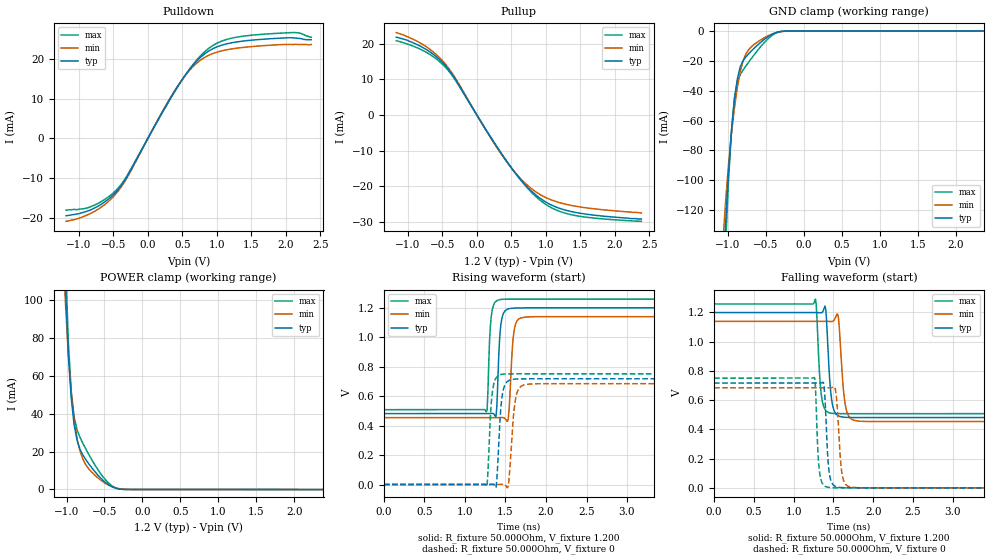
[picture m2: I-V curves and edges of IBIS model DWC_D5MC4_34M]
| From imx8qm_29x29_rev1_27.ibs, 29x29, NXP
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[Model] DWC_D5MC4_34M
Model_type   I/O
Polarity   Non-Inverting
Enable   Active-High
C_comp   1.264pF   1.181pF   1.367pF
C_comp_pullup   284.419fF   263.792fF   311.358fF
C_comp_pulldown 969.046fF   901.845fF   1.049pF
Vinh = 693.000mV
Vinl = 507.000mV
Vmeas = 600.000mV
Vref = 600.000mV
Rref = 50Ohms
Cref = 0pF
[Model Spec]
Vinh   693.000mV   663.000mV   723.000mV
Vinl   507.000mV   477.000mV   537.000mV
Vmeas   600.000mV   570.000mV   630.000mV
Vref   600.000mV   570.000mV   630.000mV
D_overshoot_ampl_h 0.4 NA   NA
D_overshoot_ampl_l 0.4 NA   NA
D_overshoot_area_l 60.000p NA   NA
D_overshoot_area_h 60.000p NA   NA
[Receiver Thresholds]
Vth = 600.000mV
Vth_min = 588.000mV
Vth_max = 612.000mV
Vinh_ac = 68.000mV
Vinh_dc = 68.000mV
Vinl_ac = -68.000mV
Vinl_dc = -68.000mV
Tslew_ac = 5.000ns
Reference_supply Pullup_ref
[Temperature Range]   25.000   125.000   -40.000
[Voltage Range]   1.200V   1.140V   1.260V
[GND Clamp Reference]   0.00V   0.00V   0.00V
[C Comp Corner]
| variable   typ   min   max
C_comp 1.264pF   1.367pF   1.181pF
C_comp_pullup 284.419fF   311.358fF   263.792fF
C_comp_pulldown 969.046fF   1.049pF   901.845fF
[Pulldown Reference]   0.00V   0.00V   0.00V
[POWER Clamp Reference]   1.200V   1.140V   1.260V
[Pullup Reference]   1.200V   1.140V   1.260V
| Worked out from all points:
|   slope of the pulldown table from 0 to 0.18 V, typ, clamps not added: 31.8 ohm
|   slope of the pullup table from 0 to 0.18 V, typ, clamps not added: 31.9 ohm
|   GND clamp passes 1 mA (typ) near -0.36 V on its own axis
|   POWER clamp passes 1 mA (typ) near -0.38 V on its own axis
|   rising waveform, R_fixture 50.000Ohm, V_fixture 1.200: 20-80 % time 37.2ps typ, 43.2ps min, 34.2ps max; typ from 0.481 V to 1.2 V
|   rising waveform, R_fixture 50.000Ohm, V_fixture 0: 20-80 % time 47.7ps typ, 56.6ps min, 43.8ps max; typ from 0 V to 0.717 V
|   falling waveform, R_fixture 50.000Ohm, V_fixture 1.200: 20-80 % time 50.4ps typ, 57.6ps min, 46.1ps max; typ from 1.2 V to 0.481 V
|   falling waveform, R_fixture 50.000Ohm, V_fixture 0: 20-80 % time 41.8ps typ, 50ps min, 36.8ps max; typ from 0.717 V to 0 V
[GND Clamp]
-1.184V   -342.5mA   -256.9mA   -430.7mA
-1.069V   -170mA     -142.2mA   -199.2mA
-1.031V   -127.6mA   -113.2mA   -142.7mA
-992.7mV  -93.59mA   -88.73mA   -98.99mA
-954.5mV  -66.78mA   -68.42mA   -66.61mA
-916.4mV  -46.35mA   -51.62mA   -45.02mA
-878.2mV  -32.2mA    -37.95mA   -34mA
-840mV    -24.05mA   -27.38mA   -29.18mA
-763.6mV  -17.22mA   -15.2mA    -23.29mA
-610.9mV  -9.369mA   -7.283mA   -12.96mA
-267.3mV  -89.24uA   -208uA     -59.9uA
2.367V    136.8uA    111.6uA    170.5uA
[Power Clamp]
-1.167V   370mA      273mA      475mA
-1.015V   108.4mA    99.12mA    123mA
-976.4mV  71.8mA     71.42mA    77.9mA
-938.2mV  48.37mA    51.03mA    51.81mA
-900mV    34.2mA     36.79mA    38.28mA
-861.8mV  25.98mA    27.04mA    31.54mA
-823.6mV  21.25mA    20.48mA    27.58mA
-747.3mV  15.81mA    13.12mA    21.46mA
-518.2mV  4.768mA    4.041mA    6.612mA
-403.6mV  1.471mA    1.528mA    1.982mA
-250.9mV  45.63uA    138.2uA    40.3uA
2.384V    -68.4uA    -58.87uA   -80.92uA
[Pulldown]
-1.184V   -19.4mA    -20.8mA    -18mA
-801.8mV  -17.73mA   -18.59mA   -16.96mA
-572.7mV  -15.26mA   -15.86mA   -14.7mA
-420mV    -12.62mA   -12.99mA   -12.28mA
-267.3mV  -8.551mA   -8.851mA   -8.351mA
381.8mV   11.65mA    11.8mA     11.55mA
572.7mV   16.61mA    16.47mA    16.66mA
763.6mV   20.38mA    19.67mA    20.77mA
992.7mV   22.94mA    21.63mA    23.84mA
1.298V    24.27mA    22.7mA     25.47mA
2.138V    25.23mA    23.63mA    26.6mA
2.367V    24.8mA     23.6mA     25.4mA
[Pullup]
-1.167V   21.8mA     23.09mA    20.81mA
-747.3mV  18.52mA    19.32mA    17.72mA
-441.8mV  13.53mA    13.94mA    13.1mA
-289.1mV  9.344mA    9.662mA    9.11mA
92.7mV    -2.936mA   -3.019mA   -2.889mA
360mV     -10.99mA   -11.12mA   -10.92mA
589.1mV   -17.07mA   -16.9mA    -17.13mA
818.2mV   -21.84mA   -21.07mA   -22.22mA
1.047V    -24.95mA   -23.59mA   -25.67mA
1.315V    -26.86mA   -25.17mA   -27.74mA
1.696V    -28.12mA   -26.34mA   -28.93mA
2.384V    -29.2mA    -27.5mA    -29.84mA
[Ramp]
R_load=50.000Ohm
dV/dt_r   430.380mV/43.000ps  410.819mV/51.000ps  450.330mV/40.000ps
dV/dt_f   430.380mV/46.500ps  410.819mV/54.500ps  450.330mV/42.000ps
[Rising waveform]
R_fixture=50.000Ohm
V_fixture=1.200
V_fixture_min=1.140
V_fixture_max=1.260
0s        481.2mV    453.7mV    507.9mV
1.263ns   481.2mV    453.7mV    493.5mV
1.273ns   481.1mV    453.7mV    507.8mV
1.323ns   482mV      453.7mV    1.135V
1.383ns   463.6mV    453.6mV    1.243V
1.444ns   1.09V      455mV      1.256V
1.534ns   1.192V     445.6mV    1.258V
1.614ns   1.197V     1.067V     1.258V
1.744ns   1.199V     1.136V     1.258V
10ns      1.199V     1.139V     1.258V
[Rising waveform]
R_fixture=50.000Ohm
V_fixture=0
0s        168.4nV    4.199uV    19.87nV
1.263ns   -5.672uV   3.087uV    -14.14mV
1.283ns   -87.45uV   5.847uV    80.13mV
1.323ns   717.7uV    19.35uV    542.9mV
1.383ns   -19.03mV   -102.7uV   722.8mV
1.464ns   619.1mV    1.652mV    748.3mV
1.534ns   703.6mV    -9.706mV   750.7mV
1.634ns   715.8mV    606.8mV    751.1mV
1.764ns   717.1mV    679.8mV    751.1mV
10ns      717.1mV    684.1mV    750.8mV
[Falling waveform]
R_fixture=50.000Ohm
V_fixture=1.200
V_fixture_min=1.140
V_fixture_max=1.260
0s        1.199V     1.139V     1.258V
1.273ns   1.199V     1.139V     1.291V
1.343ns   1.198V     1.139V     656.5mV
1.403ns   1.224V     1.139V     529.5mV
1.474ns   614.7mV    1.138V     510.5mV
1.554ns   495mV      1.188V     507.8mV
1.624ns   483.8mV    677.8mV    507.5mV
1.654ns   482.4mV    551.5mV    507.5mV
1.794ns   481mV      458mV      507.5mV
10ns      481.1mV    453.7mV    507.8mV
[Falling waveform]
R_fixture=50.000Ohm
V_fixture=0
0s        717mV      684.1mV    750.7mV
1.263ns   717mV      684.1mV    753mV
1.303ns   716.9mV    684.1mV    259.7mV
1.323ns   716.6mV    684.1mV    116.1mV
1.383ns   689.7mV    684.1mV    15.17mV
1.444ns   115mV      683.6mV    2.713mV
1.524ns   10.26mV    675.3mV    323.1uV
1.614ns   1.426mV    76.69mV    30.89uV
1.734ns   122uV      4.34mV     5.913uV
10ns      304.4nV    4.365uV    217.4nV
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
